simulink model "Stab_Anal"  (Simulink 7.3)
settings: Solver=ode45  StartTime=0.0  StopTime=500  RelTol=1e-3
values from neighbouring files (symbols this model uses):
  Ave = [    [vehicle_sim.m]
  Bve = [    [vehicle_sim.m]
  Cve = [    [vehicle_sim.m]
  Dve = [    [vehicle_sim.m]
undefined symbols (not defined in the file or in its folder): Kmix, Kpr, Kq

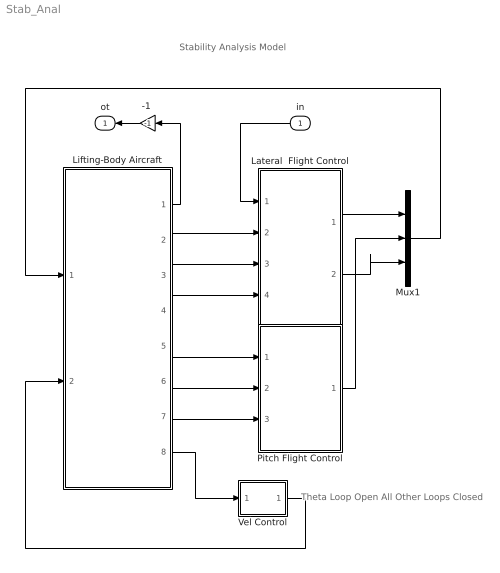
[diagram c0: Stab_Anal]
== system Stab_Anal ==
  note: Stability Analysis Model
  note: Theta Loop Open All Other Loops Closed
  in : Inport  OutDataType=sfix(16)  OutScaling=2^0
  "-1 " : Gain  Gain=-1  ParameterDataType=sfix(16)  ParameterScaling=2^0  OutDataType=sfix(16)  OutScaling=2^0
  Lateral  Flight Control : Subsystem
  Lifting-Body Aircraft : Subsystem
  Mux1 : Mux  Inputs=3
  Pitch Flight Control : Subsystem
  Vel Control : Subsystem
  ot : Outport  OutDataType=sfix(16)  OutScaling=2^0
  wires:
  Lifting-Body Aircraft/2(p) -> Lateral  Flight Control/2(pb)
  Lifting-Body Aircraft/3(r) -> Lateral  Flight Control/3(rb)
  Lifting-Body Aircraft/4(Ny) -> Lateral  Flight Control/4(beta)
  Lifting-Body Aircraft/6(q) -> Pitch Flight Control/2(q)
  Lifting-Body Aircraft/7(Nz) -> Pitch Flight Control/3(Nz)
  "-1 "/1 -> ot/1
  Vel Control/1(ax) -> Lifting-Body Aircraft/2(Ax)
  Mux1/1 -> Lifting-Body Aircraft/1(PQR dem)
  Lateral  Flight Control/1(dP) -> Mux1/1
  Lateral  Flight Control/2(dR) -> Mux1/3
  Pitch Flight Control/1(dQ) -> Mux1/2
  Lifting-Body Aircraft/8(Vd) -> Vel Control/1(Vdot)
  Lifting-Body Aircraft/5(thet) -> Pitch Flight Control/1(theta)
  Lifting-Body Aircraft/1(phi) -> "-1 "/1
  in/1 -> Lateral  Flight Control/1(phi)

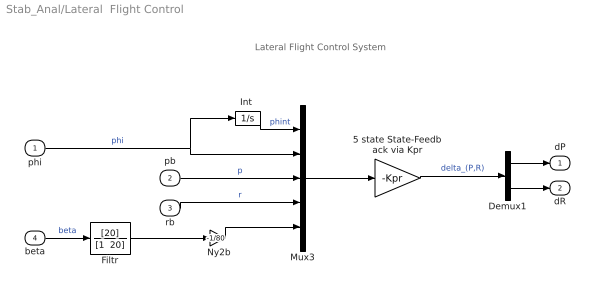
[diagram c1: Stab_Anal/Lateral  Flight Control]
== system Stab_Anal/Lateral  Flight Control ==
  note: Lateral Flight Control System
  phi : Inport  OutDataType=sfix(16)  OutScaling=2^0
  pb : Inport  Port=2  OutDataType=sfix(16)  OutScaling=2^0
  rb : Inport  Port=3  OutDataType=sfix(16)  OutScaling=2^0
  beta : Inport  Port=4  OutDataType=sfix(16)  OutScaling=2^0
  " Ny2b" : Gain  Gain=-1/80  ParameterDataType=sfix(16)  ParameterScaling=2^0  OutDataType=sfix(16)  OutScaling=2^0
  5 state State-Feedback via Kpr : Gain  Gain=-Kpr  Multiplication=Matrix(K*u)  ParameterDataType=sfix(16)  ParameterScaling=2^0  OutDataType=sfix(16)  OutScaling=2^0
  Demux1 : Demux  Outputs=2
  Filtr : TransferFcn  Numerator=[20]  Denominator="[1  20]"
  "Int " : Integrator
  Mux3 : Mux  Inputs=5
  dP : Outport  OutDataType=sfix(16)  OutScaling=2^0
  dR : Outport  Port=2  OutDataType=sfix(16)  OutScaling=2^0
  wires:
  Mux3/1 -> 5 state State-Feedback via Kpr/1
  phi/1 -> "Int "/1, Mux3/2  "phi"
  "Int "/1 -> Mux3/1  "phint"
  Demux1/2 -> dR/1
  Demux1/1 -> dP/1
  5 state State-Feedback via Kpr/1 -> Demux1/1  "delta_(P,R)"
  beta/1 -> Filtr/1  "beta"
  pb/1 -> Mux3/3  "p"
  rb/1 -> Mux3/4  "r"
  " Ny2b"/1 -> Mux3/5
  Filtr/1 -> " Ny2b"/1

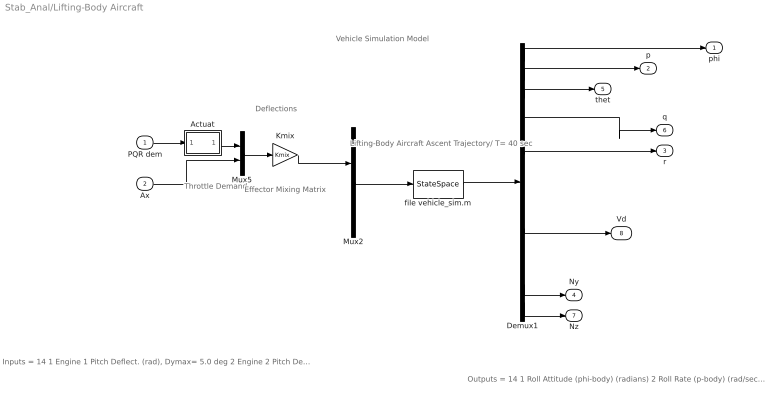
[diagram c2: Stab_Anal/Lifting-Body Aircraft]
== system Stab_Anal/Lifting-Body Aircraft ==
  note: Throttle Demand
  note: Inputs = 14 1 Engine 1 Pitch Deflect. (rad), Dymax= 5.0 deg 2 Engine 2 Pitch Deflect. (rad), Dymax= 5.0 deg 3 Engine 1 Yaw Deflection (rad), Dzmax= 5.0 deg 4 Engine 2 Yaw Deflection (rad), Dzmax= 5.0 deg 5 Throttle Input dTh/Th for Engine No1 (-) 6 Throttle Input dTh/Th for Engine No2 (-) 7 LeftElevon Deflection (radians) 8 Right Elevon Deflection (radians) 9 Vertical Rudder Deflection (radians) 10 Upper-Left Body-Flap Deflection(radians) 11 Upper-Right Body-Flap Deflection (radians) 12 Lower-Left Body-Flap Deflection(radians) 13 Lower-Right Body-Flap Deflection (radians) 14 Wind Gust Azim, Elev Angles=(45,90) (deg)
  note: Lifting-Body Aircraft Ascent Trajectory/ T= 40 sec
  note: Effector Mixing Matrix
  note: Outputs = 14 1 Roll Attitude (phi-body) (radians) 2 Roll Rate (p-body) (rad/sec) 3 Pitch Attitude (thet-bdy) (radians) 4 Pitch Rate (q-body) (rad/sec) 5 Yaw Attitude (psi-body) (radians) 6 Yaw Rate (r-body) (rad/sec) 7 Angle of attack, alfa, (radians) 8 Angle of sideslip, beta, (radian) 9 Change in Altitude, delta-h, (feet) 10 Forward Acceleration (V-dot) (ft/sec) 11 Cross Range Velocity (Vcr) (ft/sec) 12 CG Acceleration along X axis, (ft/sec^2) 13 CG Acceleration along Y axis, (ft/sec^2) 14 CG Acceleration along Z axis, (ft/sec^2)
  note: Vehicle Simulation Model
  note: Deflections
  PQR dem : Inport  OutDataType=sfix(16)  OutScaling=2^0
  Ax : Inport  Port=2  OutDataType=sfix(16)  OutScaling=2^0
  Actuat : Subsystem
  Demux1 : Demux  Outputs=14
  Kmix : Gain  Gain=Kmix  Multiplication=Matrix(K*u)  ParameterDataType=sfix(16)  ParameterScaling=2^0  OutDataType=sfix(16)  OutScaling=2^0
  Mux2 : Mux  Inputs=[13, 1]
  Mux5 : Mux  Inputs=[3, 1]
  file vehicle_sim.m : StateSpace  A=Ave  B=Bve  C=Cve  D=Dve
  phi : Outport  OutDataType=sfix(16)  OutScaling=2^0
  p : Outport  Port=2  OutDataType=sfix(16)  OutScaling=2^0
  r : Outport  Port=3  OutDataType=sfix(16)  OutScaling=2^0
  Ny : Outport  Port=4  OutDataType=sfix(16)  OutScaling=2^0
  thet : Outport  Port=5  OutDataType=sfix(16)  OutScaling=2^0
  q : Outport  Port=6  OutDataType=sfix(16)  OutScaling=2^0
  Nz : Outport  Port=7  OutDataType=sfix(16)  OutScaling=2^0
  Vd : Outport  Port=8  OutDataType=sfix(16)  OutScaling=2^0
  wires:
  Mux5/1 -> Kmix/1
  Ax/1 -> Mux5/2
  Actuat/1(ou) -> Mux5/1
  Demux1/3 -> thet/1
  Demux1/14 -> Nz/1
  Demux1/10 -> Vd/1
  file vehicle_sim.m/1 -> Demux1/1
  Demux1/1 -> phi/1
  PQR dem/1 -> Actuat/1(in)
  Demux1/6 -> r/1
  Demux1/4 -> q/1
  Demux1/2 -> p/1
  Kmix/1 -> Mux2/1
  Mux2/1 -> file vehicle_sim.m/1
  Demux1/13 -> Ny/1

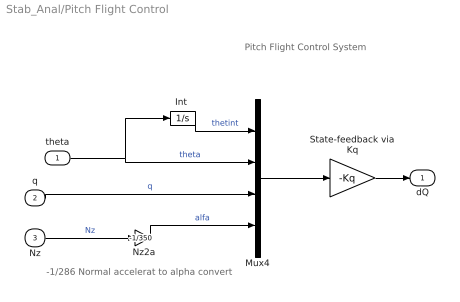
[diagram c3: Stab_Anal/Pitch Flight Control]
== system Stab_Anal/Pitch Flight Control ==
  note: -1/286 Normal accelerat to alpha convert
  note: Pitch Flight Control System
  theta : Inport  OutDataType=sfix(16)  OutScaling=2^0
  q : Inport  Port=2  OutDataType=sfix(16)  OutScaling=2^0
  Nz : Inport  Port=3  OutDataType=sfix(16)  OutScaling=2^0
  " Nz2a" : Gain  Gain=-1/350  ParameterDataType=sfix(16)  ParameterScaling=2^0  OutDataType=sfix(16)  OutScaling=2^0
  "Int " : Integrator
  Mux4 : Mux
  State-feedback via Kq : Gain  Gain=-Kq  Multiplication=Matrix(K*u)  ParameterDataType=sfix(16)  ParameterScaling=2^0  OutDataType=sfix(16)  OutScaling=2^0
  dQ : Outport  OutDataType=sfix(16)  OutScaling=2^0
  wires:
  Mux4/1 -> State-feedback via Kq/1
  theta/1 -> "Int "/1, Mux4/2  "theta"
  "Int "/1 -> Mux4/1  "thetint"
  State-feedback via Kq/1 -> dQ/1
  Nz/1 -> " Nz2a"/1  "Nz"
  " Nz2a"/1 -> Mux4/4  "alfa"
  q/1 -> Mux4/3  "q"

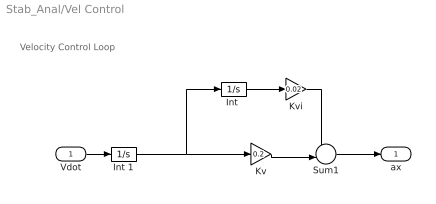
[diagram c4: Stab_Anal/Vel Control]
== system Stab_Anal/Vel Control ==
  note: Velocity Control Loop
  Vdot : Inport
  "Int " : Integrator
  Int 1 : Integrator
  Kv : Gain  Gain=0.2  ParameterDataType=fixdt(1, 16)  ParameterScaling=2^0  OutDataType=fixdt(1, 16)  OutScaling=2^0
  Kvi : Gain  Gain=0.02  ParameterDataType=fixdt(1, 16)  ParameterScaling=2^0  OutDataType=fixdt(1, 16)  OutScaling=2^0
  Sum1 : Sum  Inputs=--|  OutDataType=fixdt(1, 16)  OutScaling=2^0
  ax : Outport
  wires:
  Int 1/1 -> "Int "/1, Kv/1
  Vdot/1 -> Int 1/1
  Sum1/1 -> ax/1
  Kvi/1 -> Sum1/1
  Kv/1 -> Sum1/2
  "Int "/1 -> Kvi/1

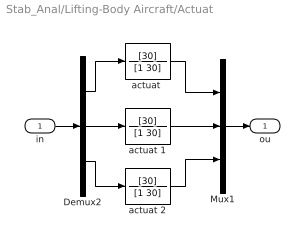
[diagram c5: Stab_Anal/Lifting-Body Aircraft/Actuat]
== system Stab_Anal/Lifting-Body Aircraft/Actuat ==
  in : Inport
  Demux2 : Demux  Outputs=3
  Mux1 : Mux  Inputs=3
  "actuat " : TransferFcn  Numerator=[30]  Denominator=[1 30]
  actuat 1 : TransferFcn  Numerator=[30]  Denominator=[1 30]
  actuat 2 : TransferFcn  Numerator=[30]  Denominator=[1 30]
  ou : Outport
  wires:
  Mux1/1 -> ou/1
  in/1 -> Demux2/1
  Demux2/3 -> actuat 2/1
  Demux2/1 -> "actuat "/1
  Demux2/2 -> actuat 1/1
  actuat 2/1 -> Mux1/3
  "actuat "/1 -> Mux1/1
  actuat 1/1 -> Mux1/2
